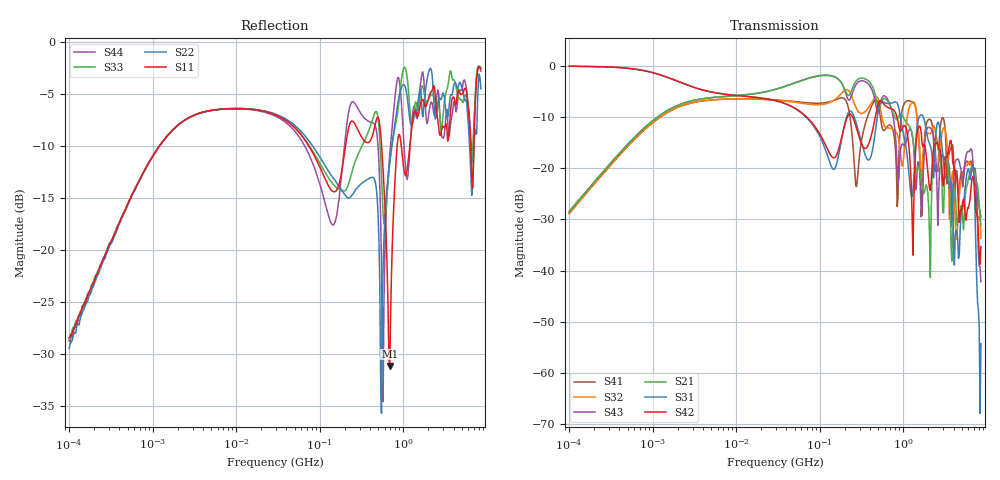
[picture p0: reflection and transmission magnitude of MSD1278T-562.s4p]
# MHz S MA R 50
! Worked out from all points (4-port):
!   498 points, 100 kHz to 8.5 GHz, reference 50 ohm
!   strongest paths, dB at 100 kHz, 1.698 MHz, 29.49 MHz, 500.7 MHz, 8.5 GHz:
!     S42: -0.1, -2.6, -6.8, -7.5, -35.3
!     S31: -0.1, -2.6, -6.8, -8.9, -54.3
!     S21: -28.5, -8.2, -4.6, -8.1, -31.2
!     S43: -28.4, -8.3, -4.6, -9.2, -42.2
!     S32: -28.8, -8.6, -6.7, -6.4, -33.7
!     S41: -28.8, -8.6, -6.6, -7.3, -29.5
!   lowest |S11| = -31.1 dB at 689.3 MHz (marker M1), VSWR 1.06, Z = 51.7 - j2.25 ohm
!   |S11| at or under -10 dB: 550.7 MHz to 845.7 MHz (295 MHz wide, 42.3 % of centre); 947 MHz to 1.199 GHz (251.6 MHz wide, 23.5 % of centre); 6.423 GHz to 7.018 GHz (594.9 MHz wide, 8.85 % of centre)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
0.1  0.03799 81.2  0.03755 83.7  0.9903 -2.2  0.03616 -96.4
     0.03755 83.7  0.03369 85.2  0.03623 -96.4  0.9918 -2.2
     0.9903 -2.2  0.03623 -96.4  0.03732 83.2  0.03783 83.7
     0.03616 -96.4  0.9918 -2.2  0.03783 83.7  0.03682 86.8
8.208072  0.4765 0.9  0.5052 13.1  0.5219 -17.0  0.4735 178.3
          0.5052 13.1  0.4766 2.8  0.4738 -179.9  0.5228 -17.0
          0.5219 -17.0  0.4738 -179.9  0.4769 2.8  0.5053 13.1
          0.4735 178.3  0.5228 -17.0  0.5053 13.1  0.4752 1.0
500.661  0.4338 -65.5  0.3956 -95.8  0.3579 67.7  0.4291 -53.1
         0.3956 -95.8  0.1448 -77.7  0.4788 -67.7  0.4229 26.1
         0.3579 67.7  0.4788 -67.7  0.4269 -50.8  0.345 -91.3
         0.4291 -53.1  0.4229 26.1  0.345 -91.3  0.3084 -102.3
689.2879  0.02772 -51.8  0.4163 -119.0  0.4286 -42.7  0.2645 -70.6
          0.4163 -119.0  0.2678 4.3  0.2469 -93.7  0.3853 -64.1
          0.4286 -42.7  0.2469 -93.7  0.2601 -24.1  0.4244 -136.5
          0.2645 -70.6  0.3853 -64.1  0.4244 -136.5  0.2864 -10.7
2110.57  0.5663 -160.9  0.008569 -147.3  0.1656 113.3  0.2987 138.9
         0.008569 -147.3  0.7461 -173.5  0.2182 151.9  0.06071 -22.7
         0.1656 113.3  0.2182 151.9  0.551 -167.3  0.2468 136.3
         0.2987 138.9  0.06071 -22.7  0.2468 136.3  0.5018 -164.6
6764.496  0.1986 109.4  0.09696 35.0  0.1061 18.1  0.09906 35.6
          0.09696 35.0  0.1987 71.8  0.0928 59.6  0.0829 49.0
          0.1061 18.1  0.0928 59.6  0.2905 100.7  0.1284 6.3
          0.09906 35.6  0.0829 49.0  0.1284 6.3  0.2857 135.4
8500  0.7404 -51.6  0.02751 -109.7  0.001933 64.8  0.03337 -148.8
      0.02751 -109.7  0.5946 -44.3  0.02072 -162.8  0.01719 -176.4
      0.001933 64.8  0.02072 -162.8  0.748 -49.3  0.007785 -36.4
      0.03337 -148.8  0.01719 -176.4  0.007785 -36.4  0.7208 -48.2
